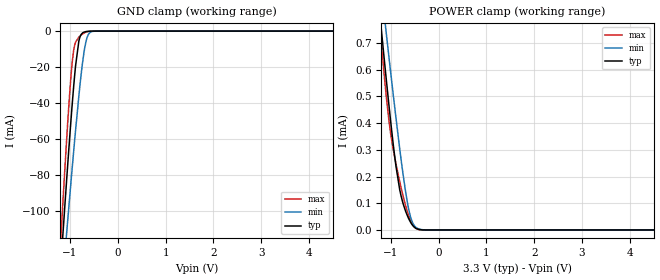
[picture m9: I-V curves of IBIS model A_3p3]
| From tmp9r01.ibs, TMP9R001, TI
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|   Model
[Model]   A_3p3
Model_type   Input
Vinl = 0.99
Vinh = 2.31
|   typ   min   max
C_comp   0.794pF   0.780pF   0.806pF
[Voltage Range]   3.3   2.7   3.6
[Temperature Range]   25   125   -40
[Power Clamp Reference]   3.3   2.7   3.6
[GND Clamp Reference]   0   0   0
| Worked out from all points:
|   GND clamp passes 1 mA (typ) near -0.73 V on its own axis
|   POWER clamp passes 1 mA (typ) near -1.33 V on its own axis
[GND Clamp]
|   Voltage   I(typ)   I(min)   I(max)
-3.3V     -1.016A    -872.1mA   -1.168A
-1.181V   -125.8mA   -148mA     -110.1mA
-1.122V   -102.5mA   -128.7mA   -82.96mA
-1.063V   -79.74mA   -109.8mA   -56.94mA
-1.003V   -57.81mA   -91.12mA   -33.21mA
-953.7mV  -40.56mA   -75.91mA   -17.24mA
-904.2mV  -24.95mA   -61.12mA   -7.97mA
-815.1mV  -5.622mA   -36.14mA   -3.379mA
-706.2mV  -588.7uA   -11.63mA   -1.1mA
-617.1mV  -113.5uA   -2.001mA   -248.7uA
-468.6mV  -4.143uA   -37.89uA   -6.719uA
6.6V      0A         0A         0A
[POWER Clamp]
|   Voltage   I(typ)   I(min)   I(max)
-3.3V     4.831mA    4.465mA    5.542mA
-1.27V    880.3uA    1.019mA    848.8uA
-1.152V   662.5uA    825.3uA    603.7uA
-1.102V   574uA      745.5uA    510.6uA
-993.3mV  387.9uA    572.8uA    347.4uA
-894.3mV  239.3uA    420.5uA    248.1uA
-815.1mV  150.6uA    304.3uA    180.9uA
-716.1mV  82.9uA     171.9uA    107.1uA
-627mV    42.31uA    77.57uA    53.42uA
-547.8mV  17.97uA    28.3uA     20.74uA
-468.6mV  5.402uA    8.675uA    5.173uA
6.6V      0A         0A         0A
